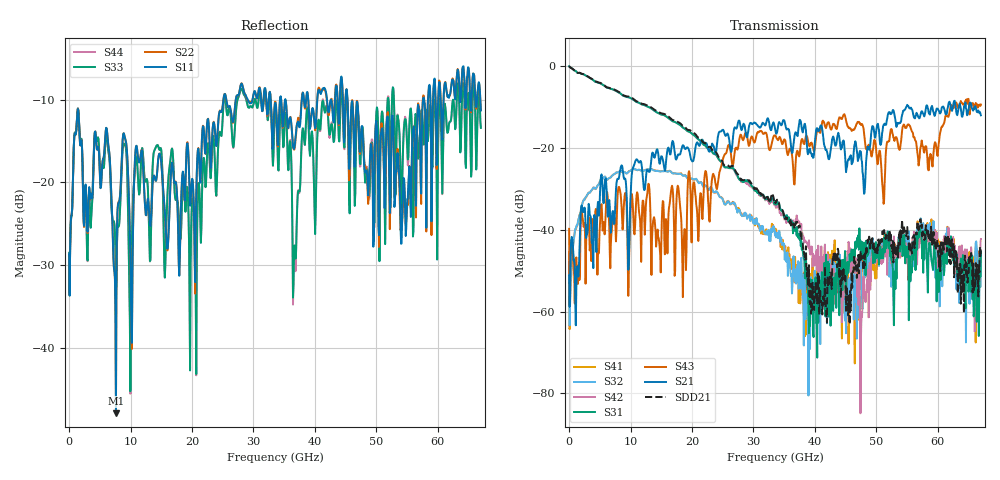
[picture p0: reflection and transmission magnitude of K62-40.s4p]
!Agilent Technologies,N5247A,US50470101,A.10.25.02
!Agilent N5247A: A.10.25.02
!Date: Tuesday, May 12, 2015 13:42:27
!Correction: Sdd11(Full 4 Port(1,2,3,4))
!Sdc11(Full 4 Port(1,2,3,4))
!Sdd12(Full 4 Port(1,2,3,4))
!Sdc12(Full 4 Port(1,2,3,4))
!Scd11(Full 4 Port(1,2,3,4))
!Scc11(Full 4 Port(1,2,3,4))
!Scd12(Full 4 Port(1,2,3,4))
!Scc12(Full 4 Port(1,2,3,4))
!Sdd21(Full 4 Port(1,2,3,4))
!Sdc21(Full 4 Port(1,2,3,4))
!Sdd22(Full 4 Port(1,2,3,4))
!Sdc22(Full 4 Port(1,2,3,4))
!Scd21(Full 4 Port(1,2,3,4))
!Scc21(Full 4 Port(1,2,3,4))
!Scd22(Full 4 Port(1,2,3,4))
!Scc22(Full 4 Port(1,2,3,4))
!Balanced Topology: BBAL
!S4P File: Measurements: <Sdd11,Sdc11,Sdd12,Sdc12>,
!<Scd11,Scc11,Scd12,Scc12>,
!<Sdd21,Sdc21,Sdd22,Sdc22>,
!<Scd21,Scc21,Scd22,Scc22>:
# Hz S  dB  R 50
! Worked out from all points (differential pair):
!   801 points, 10 MHz to 67 GHz, reference 50 ohm
!   strongest paths, dB at 10 MHz, 16.76 GHz, 33.51 GHz, 50.25 GHz, 67 GHz:
!     S21: -51.1, -18.7, -15.2, -14.1, -12.0
!     S43: -39.8, -29.3, -16.9, -23.9, -9.4
!     S31: -0.1, -13.4, -33.3, -46.1, -45.3
!     S42: 0.0, -13.4, -33.8, -44.0, -42.3
!     S32: -47.8, -26.2, -41.4, -45.0, -45.5
!     S41: -45.5, -26.1, -39.7, -44.3, -48.1
!   taken as a pair (ports 1,2 in; 3,4 out), SDD21 dB: 0.0, -13.1, -33.0, -43.8, -44.2
!   lowest |S11| = -47.9 dB at 7.63 GHz (marker M1), VSWR 1.01, Z = 49.6 - j0.186 ohm
!   |S11| at or under -10 dB: start of sweep to 25.12 GHz; 35.21 GHz to 37.87 GHz (2.665 GHz wide, 7.29 % of centre); 45.3 GHz to 57.6 GHz (12.3 GHz wide, 23.9 % of centre)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
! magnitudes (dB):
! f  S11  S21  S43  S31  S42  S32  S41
! 10 MHz  -28.7  -51.1  -39.8  -0.1  0.0  -47.8  -45.5
! 7.63 GHz  -47.9  -30.4  -42.9  -6.1  -6.1  -26.1  -26.1
! 33.92 GHz  -15.3  -15.5  -18.0  -33.5  -34.1  -40.8  -41.5
! 39.2 GHz  -13.5  -20.2  -19.3  -63.5  -46.0  -69.1  -50.8
! 47.41 GHz  -15.2  -20.9  -14.1  -42.7  -84.9  -46.4  -47.9
! 56.78 GHz  -10.6  -12.4  -22.5  -40.8  -41.6  -39.2  -40.8
! 67 GHz  -11.3  -12.0  -9.4  -45.3  -42.3  -45.5  -48.1
